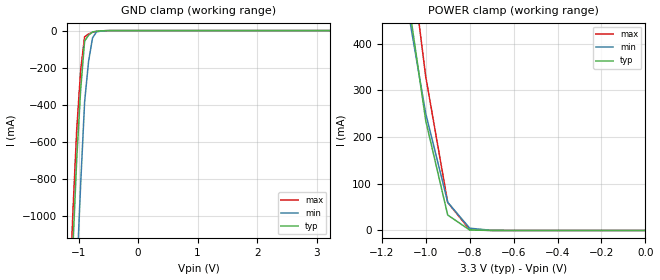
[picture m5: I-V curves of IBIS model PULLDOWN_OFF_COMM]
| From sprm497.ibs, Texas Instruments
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|   Model Cell PULLDOWN_OFF_COMM
[Model]   PULLDOWN_OFF_COMM
Model_type   Input
Polarity   Non-Inverting
Vinl =  0.8
Vinh =  2
C_comp   0.8695239p   0.8563616p   0.8781626p
[Model Spec]
Vinl   0.8   0.8   0.8
Vinh   2   2   2
[Temperature Range]   25   105   0
[Voltage Range]   3.3   3.14   3.47
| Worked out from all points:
|   GND clamp passes 1 mA (typ) near -0.58 V on its own axis
|   POWER clamp passes 1 mA (typ) near -0.80 V on its own axis
[POWER_clamp]
|   voltage   I(typ)   I(min)   I(max)
-3.3V     9.572A     8.242A     10.54A
-1.067V   452.1mA    433.2mA    579.3mA
-1.033V   343.5mA    341.6mA    454.2mA
-1V       234.9mA    250.1mA    329.1mA
-900mV    33.01mA    60.36mA    60.01mA
-800mV    1.012mA    4.898mA    1.657mA
-700mV    23.28uA    258.4uA    27.13uA
-11.55fV  368.6pA    4.318nA    659.1pA
[GND_clamp]
|   voltage   I(typ)   I(min)   I(max)
-3.3V     -22.43A    -23.04A    -22.26A
-1.167V   -1.763A    -2.446A    -1.569A
-1.1V     -1.191A    -1.863A    -1.003A
-1.033V   -696.7mA   -1.322A    -538.1mA
-966.7mV  -318.5mA   -829.3mA   -215mA
-900mV    -56.17mA   -384.9mA   -33.52mA
-833.3mV  -25.14mA   -165.5mA   -18.52mA
-766.7mV  -7.667mA   -39.43mA   -8.915mA
-700mV    -3.749mA   -6.74mA    -4.716mA
-633.3mV  -1.908mA   -3.333mA   -2.394mA
3.233V    348.5pA    4.567nA    506.4pA
